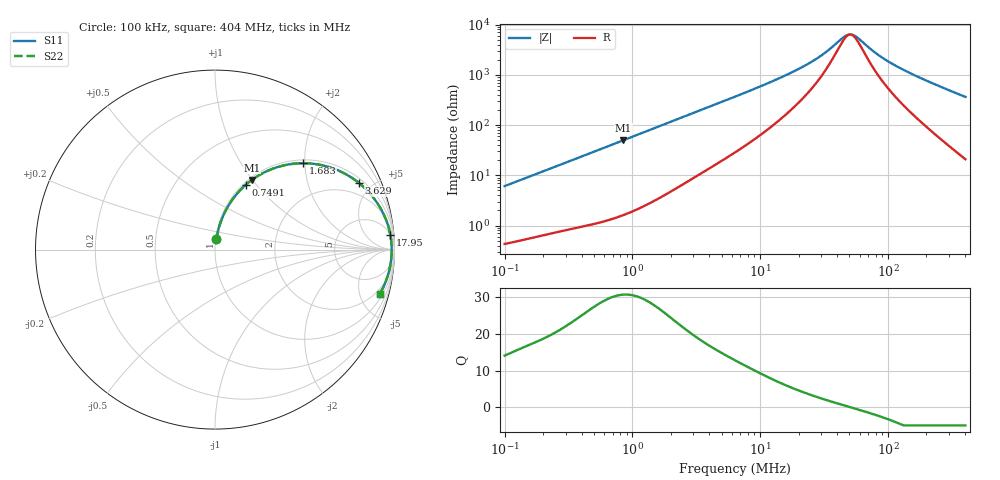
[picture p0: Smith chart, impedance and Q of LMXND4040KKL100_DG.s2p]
! LMXND4040KKL100_DG  S-PARAMETER MODEL  ( General Type )
! Model Generated by TAIYO YUDEN Corporation (http://www.ty-top.com)
! Version 1.0
! TAIYO YUDEN Control No. 191023NI43SB-FBB
! Copyright(c) 2019 TAIYO YUDEN CO.,LTD. All Rights Reserved.
! Product Description (link to TY-COMPAS)
! https://ds.yuden.co.jp/TYCOMPAS/or/detail?pn=LMXND4040KKL100MDG&u=M
! Products Name : Inductors
! Characteristics :
!  Inductance : 10 uH , SRF(min) : 31 MHz , DC Resistance(max) : 0.36 Ohm
!  Rated Current : Saturation :620 mA , Temp Rise : 750 mA
!  Case Size : 4.0 x 4.0 / 0.157 x 0.157 [mm/inch] , Thickness : 1 / 0.039 [mm/inch]
!  (Conditions: Temperature = 25 degC , DC Bias Current/Voltage = 0A / 0V)
! External Node Assignments :
!  1  o---GGG---o  2
! GND o---------o GND
! Frequency Range : 0.1MHz  -  403.964729MHz  [ 402 STEP ]
# MHz S RI R 50
! Freq[MHz].  S11 Real  S11 Imag  S21 Real  S21 Imag  S12 Real  S12 Imag  S22 Real  S22 Imag
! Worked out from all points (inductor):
!   401 points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, 100 kHz to 404 MHz, reference 50 ohm
!   read as one part in series: L = 9.65 uH near 104.2 kHz
!   highest Q = 30.8 at 848.5 kHz (marker M1), where L = 9.33 uH
!   self-resonance near 50.66 MHz
!   S11 on the Smith chart (normalised r, x): 100 kHz: 1.01, +0.12; 749.1 kHz: 1.03, +0.88; 1.683 MHz: 1.07, +1.96; 3.629 MHz: 1.24, +4.19; 17.95 MHz: 5, +22; 404 MHz: 1.42, -7.25
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0.1  0.00796 0.0602  0.992 -0.0602  0.992 -0.0602  0.00796 0.0602
0.21114  0.0221 0.123  0.9779 -0.123  0.9779 -0.123  0.0221 0.123
0.401849  0.0614 0.221  0.9386 -0.221  0.9386 -0.221  0.0614 0.221
0.749097  0.1702 0.3597  0.8298 -0.3597  0.8298 -0.3597  0.1702 0.3597
0.848464  0.2062 0.3887  0.7938 -0.3887  0.7938 -0.3887  0.2062 0.3887
1.207544  0.3382 0.4566  0.6618 -0.4566  0.6618 -0.4566  0.3382 0.4566
1.614823  0.4717 0.481  0.5283 -0.481  0.5283 -0.481  0.4717 0.481
1.683282  0.4915 0.4814  0.5085 -0.4814  0.5085 -0.4814  0.4915 0.4814
2.346446  0.6446 0.457  0.3554 -0.457  0.3554 -0.457  0.6446 0.457
3.628637  0.8019 0.3714  0.1981 -0.3714  0.1981 -0.3714  0.8019 0.3714
6.355822  0.9147 0.2431  0.0853 -0.2431  0.0853 -0.2431  0.9147 0.2431
11.13269  0.9613 0.1425  0.0387 -0.1425  0.0387 -0.1425  0.9613 0.1425
17.94588  0.9767 0.0829  0.0233 -0.0829  0.0233 -0.0829  0.9767 0.0829
25.54079  0.9816 0.05  0.0184 -0.05  0.0184 -0.05  0.9816 0.05
32.76608  0.9834 0.0304  0.0166 -0.0304  0.0166 -0.0304  0.9834 0.0304
44.73654  0.9844 0.00845  0.0156 -0.00845  0.0156 -0.00845  0.9844 0.00845
50.67078  0.9845 -2.08e-05  0.0155 2.08e-05  0.0155 2.08e-05  0.9845 -2.08e-05
57.39218  0.9845 -0.00849  0.0155 0.00849  0.0155 0.00849  0.9845 -0.00849
78.35931  0.9836 -0.0305  0.0164 0.0305  0.0164 0.0305  0.9836 -0.0305
102.6353  0.9818 -0.0519  0.0182 0.0519  0.0182 0.0519  0.9818 -0.0519
183.5443  0.9716 -0.1121  0.0284 0.1121  0.0284 0.1121  0.9716 -0.1121
403.9647  0.9173 -0.2481  0.0827 0.2481  0.0827 0.2481  0.9173 -0.2481
